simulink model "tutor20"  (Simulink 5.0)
settings: Solver=ode45  SolverMode=SingleTasking  StartTime=0.0  StopTime=10  RelTol=1e-3  AbsTol=1e-3
libraries: simulink x1

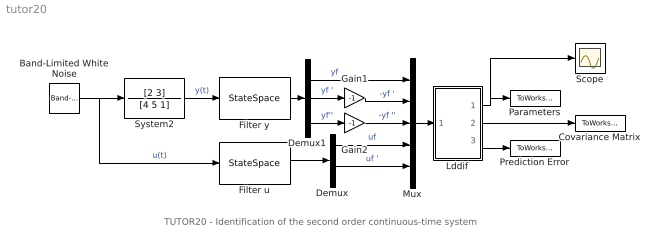
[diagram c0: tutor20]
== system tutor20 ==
  note: TUTOR20 - Identification of the second order continuous-time system
  Band-Limited White Noise : simulink/Sources/Band-Limited White Noise  Cov=[0.1]  Ts=0.1  seed=[23341]
  Covariance Matrix : ToWorkspace  VariableName=CovMatrix  SaveFormat=Array
  Demux : Demux  Outputs=2
  Demux1 : Demux  Outputs=3
  Filter u : StateSpace  A=[0 1 0;0 0 1;-1 -3 -3]  B=[0;0;1]  C=[1 0 0;0 1 0]  D=[0;0]  X0=[0 0 0]
  Filter y : StateSpace  A=[0 1 0;0 0 1;-1 -3 -3]  B=[0;0;1]  C=eye(3)  D=[0;0;0]  X0=[0 0 0]
  Gain1 : Gain  Gain=-1
  Gain2 : Gain  Gain=-1
  Lddif : Subsystem  mask(LDDIF){par=[4,1], L=[0.985], d=[0.01], poc=[0 0 0 0], kov=[10e6], ts=[1]}
      mask prompts: par "No. of estimated parameters and outputs - [n,m]:"; L "Exponential forgetting - [L]:"; d "Bittanti's correction - [d]:"; poc "Initial parameter estimates - [theta(1) ... theta(n)]:"; kov "Covariance matrix (see help, standard - [10e6]):"; ts "Sampling period - [ts]:"
      mask help: LDDIF: + Bittanti's corrections Authors: Lubos Cirka and Miroslav Fikar 1998 - 2006
      mask init:
      | n=par(1); m=par(2);
  Mux : Mux  Inputs=5
  Parameters : ToWorkspace  VariableName=BA  SaveFormat=Array
  Prediction Error : ToWorkspace  VariableName=PredError  SaveFormat=Array
  Scope : Scope
  System2 : TransferFcn  Numerator=[2 3]  Denominator=[4 5 1]
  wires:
  Band-Limited White Noise/1 -> Filter u/1, System2/1  "u(t)"
  System2/1 -> Filter y/1  "y(t)"
  Demux1/2 -> Gain1/1  "yf '"
  Filter u/1 -> Demux/1
  Demux1/3 -> Gain2/1  "yf''"
  Filter y/1 -> Demux1/1
  Mux/1 -> Lddif/1("y, z")
  Demux/2 -> Mux/5  "uf '"
  Gain2/1 -> Mux/3  "-yf ''"
  Gain1/1 -> Mux/2  "-yf '"
  Demux1/1 -> Mux/1  "yf"
  Demux/1 -> Mux/4  "uf"
  Lddif/2(covariance matrix) -> Covariance Matrix/1
  Lddif/3(prediction error) -> Prediction Error/1
  Lddif/1(theta) -> Parameters/1, Scope/1

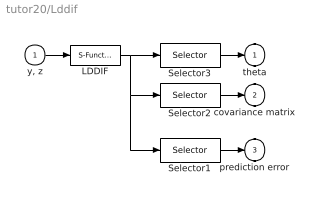
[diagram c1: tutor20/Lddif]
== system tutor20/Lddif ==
  "y, z" : Inport
  LDDIF : S-Function  FunctionName=lddif_s  Parameters=m, n, L, d, poc, kov, ts
  Selector1 : Selector  Elements=[n*m+n*n+1:1:n*m+n*n+m]  InputPortWidth=n*m+n*n+m
  Selector2 : Selector  Elements=[n*m+1:1:n*m+n*n]  InputPortWidth=n*m+n*n+m
  Selector3 : Selector  Elements=[1:1:n*m]  InputPortWidth=n*m+n*n+m
  theta : Outport  InitialOutput=0
  covariance matrix : Outport  Port=2  InitialOutput=0
  prediction error : Outport  Port=3  InitialOutput=0
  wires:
  "y, z"/1 -> LDDIF/1
  LDDIF/1 -> Selector1/1, Selector2/1, Selector3/1
  Selector2/1 -> covariance matrix/1
  Selector3/1 -> theta/1
  Selector1/1 -> prediction error/1
